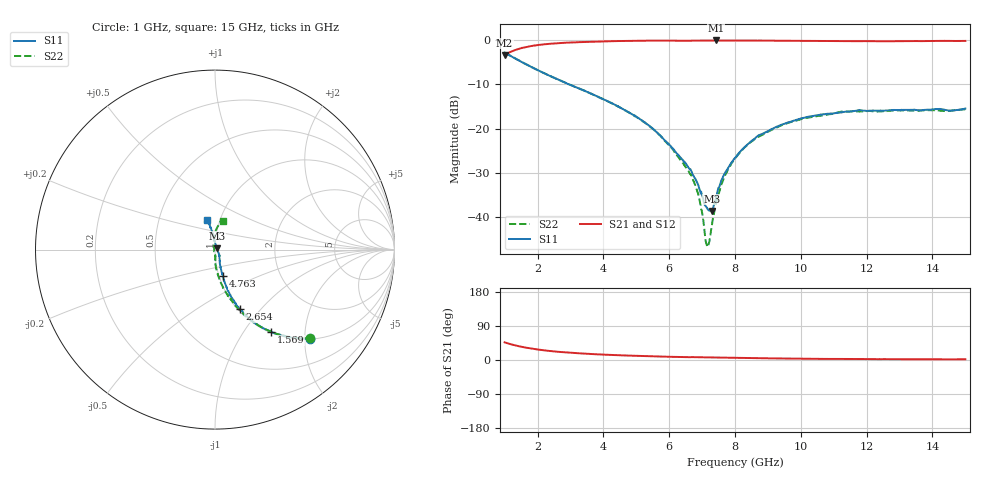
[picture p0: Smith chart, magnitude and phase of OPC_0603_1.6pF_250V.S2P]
! FILE NAME
! DATE 08/20/2012  15:27
! CORRECTED  DATA
# GHz  S  MA  R  50.00
!  FREQ  S11M  S11A  S21M  S21A  S12M  S12A  S22M  S22A
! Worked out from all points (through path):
!   1601 points, 1 GHz to 15 GHz, reference 50 ohm
!   highest |S21| = -0.05 dB at 7.423 GHz (marker M1); lowest = -3.3 dB at 1 GHz (marker M2)
!   group delay of S21, straight-line fit = 5.61 ps
!   lowest |S11| = -38.6 dB at 7.291 GHz (marker M3), VSWR 1.02, Z = 50.9 + j0.719 ohm
!   |S11| at or under -10 dB: 2.963 GHz to end of sweep
!   |S22| runs from -46.5 to -2.8 dB; largest |S21 - S12| = 0.0077
!   S11 on the Smith chart (normalised r, x): 1 GHz: 1.02, -2.12; 1.569 GHz: 1.02, -1.34; 2.654 GHz: 1.02, -0.77; 4.763 GHz: 1.04, -0.32; 15 GHz: 0.87, +0.29
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1  0.7245 -43.1  0.6814 46.6  0.6812 46.6  0.7246 -43.0
1.56875  0.555 -55.6  0.8241 33.9  0.8245 34.0  0.5549 -55.5
2.65375  0.3567 -67.4  0.9269 21.5  0.926 21.5  0.3557 -68.3
3.33625  0.2782 -71.0  0.9544 17.3  0.9539 17.3  0.2773 -73.6
4.7625  0.1538 -73.7  0.983 11.6  0.9832 11.7  0.1538 -82.5
5.6725  0.08777 -71.6  0.9902 9.2  0.9904 9.3  0.08716 -88.0
6.0925  0.06084 -64.7  0.9888 8.3  0.9883 8.3  0.05938 -88.3
6.71375  0.03046 -47.5  0.9889 7.6  0.9885 7.6  0.02718 -91.0
6.92375  0.02067 -36.0  0.9912 7.2  0.9905 7.3  0.01549 -104.7
7.09875  0.01354 -9.5  0.992 7.0  0.9916 7.0  0.005672 -138.3
7.15125  0.01275 1.0  0.9922 6.9  0.9918 7.0  0.004706 -168.5
7.2125  0.01186 16.4  0.9926 6.8  0.9921 6.8  0.005209 150.4
7.29125  0.01175 36.9  0.9933 6.7  0.9932 6.8  0.007793 125.6
7.4225  0.01664 69.1  0.9943 6.4  0.9929 6.5  0.01422 112.0
7.65  0.02938 82.9  0.9937 6.1  0.9929 6.2  0.02707 104.5
8  0.04685 91.8  0.9935 5.6  0.9928 5.7  0.04591 98.3
8.72625  0.08468 97.1  0.9912 4.8  0.9909 4.8  0.08165 90.0
9.4875  0.1133 100.2  0.9874 4.0  0.9874 4.0  0.112 86.4
10.33625  0.1387 102.1  0.9831 3.2  0.9823 3.2  0.1354 81.9
11.2375  0.1528 105.1  0.9747 2.8  0.9742 2.8  0.1559 79.4
12.6725  0.1612 109.2  0.9722 2.4  0.9723 2.4  0.1588 76.4
15  0.1692 105.2  0.9826 2.1  0.9822 2.1  0.1667 74.9
